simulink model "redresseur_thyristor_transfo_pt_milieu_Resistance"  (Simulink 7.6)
settings: Solver=ode23tb  StartTime=0.0  StopTime=1  RelTol=1e-4
InitFcn:
  | clear all, close all, clc
  | N=0.1;
StopFcn:
  | close all
  | load Iak_Vak.mat
  | 
  | subplot(2,1,1)
  | plotyy(x(1,:),x(2,:), x(1,:),x(3,:))
  | grid
  | title('Courant Iak et tension Vak du Thyristor1')
  | xlabel('temps')
  | 
  | subplot(2,1,2)
  | plotyy(x(1,:),x(4,:), x(1,:),x(5,:))
  | grid
  | title('Courant Iak et tension Vak du Thyristor2')
  | xlabel('temps')
  | 
  | figure(2)
  | load Vs.mat
  | plot(y(1,:),y(2,:))
  | grid
  | title('Tension aux bornes de la résistance R de charge')
  | xlabel('temps')
  | axis([0 1 0 70])
libraries: powerlib x9

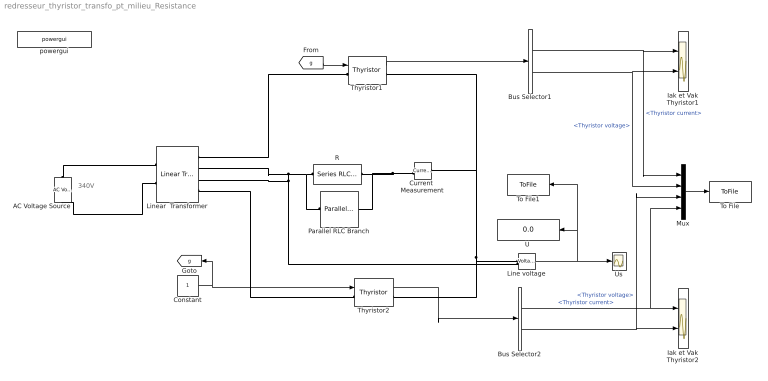
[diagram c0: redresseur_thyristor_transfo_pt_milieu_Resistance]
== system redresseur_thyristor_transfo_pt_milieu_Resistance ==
  note: 340V
  AC Voltage Source : powerlib/Electrical Sources/AC Voltage Source  DialogController=POWERSYS.PowerSysDialog  SystemSampleTime=-1  Amplitude=220  Phase=0  Frequency=60  SampleTime=0  Measurements=None
  Bus Selector1 : BusSelector  OutputSignals=Thyristor current,Thyristor voltage
  Bus Selector2 : BusSelector  OutputSignals=Thyristor current,Thyristor voltage
  Constant : Constant
  Current  Measurement : powerlib/Measurements/Current Measurement  DialogController=POWERSYS.PowerSysDialog  SystemSampleTime=-1  PhasorSimulation=off  OutputType=Complex  PSBequivalent=0
  Iak et Vak Thyristor1 : Scope  NumInputPorts=2
  Iak et Vak Thyristor2 : Scope  NumInputPorts=2
  Line voltage : powerlib/Measurements/Voltage Measurement  Tag=PoWeRsYsTeMmEaSuReMeNt  DialogController=POWERSYS.PowerSysDialog  SystemSampleTime=-1  PhasorSimulation=off  OutputType=Magnitude  PSBequivalent=0
  Linear  Transformer : powerlib/Elements/Linear Transformer  DialogController=POWERSYS.PowerSysDialog  PhysicalDomain=powersysdomain  SubClassName=unknown  LeftPortType=p1  RightPortType=p1  LConnTagsString=a|b  RConnTagsString=A|B|C|D  UNITS=pu  NominalPower="[500  60 ]"  winding1="[ 500  0.002  0.08 ]"  winding2="[250  0.002  0.08 ]"  ThreeWindings=on  winding3=[ 250 0.002 0.08 ]  RmLm=[ 500 500 ]  Measurements=None  DataType=off
  Mux : Mux
  Parallel RLC Branch : powerlib/Elements/Parallel RLC Branch  DialogController=POWERSYS.PowerSysDialog  PhysicalDomain=powersysdomain  SubClassName=unknown  LeftPortType=p1  RightPortType=p1  LConnTagsString=a  RConnTagsString=__new0  BranchType=C  Resistance=1  Inductance=1e-3  SetiL0=off  InitialCurrent=0  Capacitance=10e-3  Setx0=off  InitialVoltage=0  Measurements=None
  R : powerlib/Elements/Series RLC Branch  DialogController=POWERSYS.PowerSysDialog  PhysicalDomain=powersysdomain  SubClassName=unknown  LeftPortType=p1  RightPortType=p1  LConnTagsString=__new0  RConnTagsString=__new0  BranchType=R  Resistance=47  Inductance=1e-3  SetiL0=off  InitialCurrent=0  Capacitance=1e-6  Setx0=off  InitialVoltage=0  Measurements=None
  Thyristor1 : powerlib/Power Electronics/Thyristor  DialogController=POWERSYS.PowerSysDialog  SystemSampleTime=-1  Ron=0.001  Lon=0  Vf=0.8  IC=0  Rs=500  Cs=250e-9  Measurements=on
  Thyristor2 : powerlib/Power Electronics/Thyristor  DialogController=POWERSYS.PowerSysDialog  SystemSampleTime=-1  Ron=0.001  Lon=0  Vf=0.8  IC=0  Rs=500  Cs=250e-9  Measurements=on
  To File : ToFile  Filename=Iak_Vak  MatrixName=x
  To File1 : ToFile  Filename=Vs  MatrixName=y
  "U " : Display
  Us : Scope
  powergui : powerlib/powergui  Priority=1  SystemSampleTime=-1  SimulationMode=Continuous  SampleTime=50e-6  frequency=60  SPID=off  DisableSnubberDevices=off  DisableRonSwitches=off  DisableVfSwitches=off  SwTol=0  Interpol=off  frequencyindice=0  echomessages=off  HookPort=off  DisplayEquations=off  FunctionMessages=off  EnableUseOfTLC=off  x0status=blocks  RestoreLinks=warning  ResistiveCurrentMeasurement=off  Ylog=off  Xlog=on  ShowGrid=off  save=off  variable=ZData  ZoomFFT=off  StartTime=0.0  cycles=1  DisplayStyle=1  fundamental=60  FreqAxis=off  MaxFrequency=1000  frequencyindicesteady=1  display=off  methode=off
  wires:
  Constant/1 -> Thyristor2/1, [g]
  [g] -> Thyristor1/1
  Line voltage/1 -> Us/1, "U "/1, To File1/1
  Thyristor1/1 -> Bus Selector1/1
  Thyristor2/1 -> Bus Selector2/1
  Bus Selector2/1 -> Iak et Vak Thyristor2/1, Mux/4  "<Thyristor current>"
  Bus Selector1/1 -> Iak et Vak Thyristor1/1, Mux/1  "<Thyristor current>"
  Bus Selector1/2 -> Iak et Vak Thyristor1/2, Mux/2  "<Thyristor voltage>"
  Bus Selector2/2 -> Iak et Vak Thyristor2/2, Mux/3  "<Thyristor voltage>"
  Mux/1 -> To File/1
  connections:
  Linear  Transformer/LConn2 -- AC Voltage Source/LConn1
  AC Voltage Source/RConn1 -- Linear  Transformer/LConn1
  Linear  Transformer/RConn4 -- Thyristor2/LConn1
  Thyristor1/LConn1 -- Linear  Transformer/RConn1
  Thyristor2/RConn1 -- Line voltage/LConn1 -- Thyristor1/RConn1 -- Current  Measurement/LConn1
  R/LConn1 -- Linear  Transformer/RConn3 -- Line voltage/LConn2 -- Linear  Transformer/RConn2 -- Parallel RLC Branch/LConn1
  Current  Measurement/RConn1 -- R/RConn1 -- Parallel RLC Branch/RConn1
